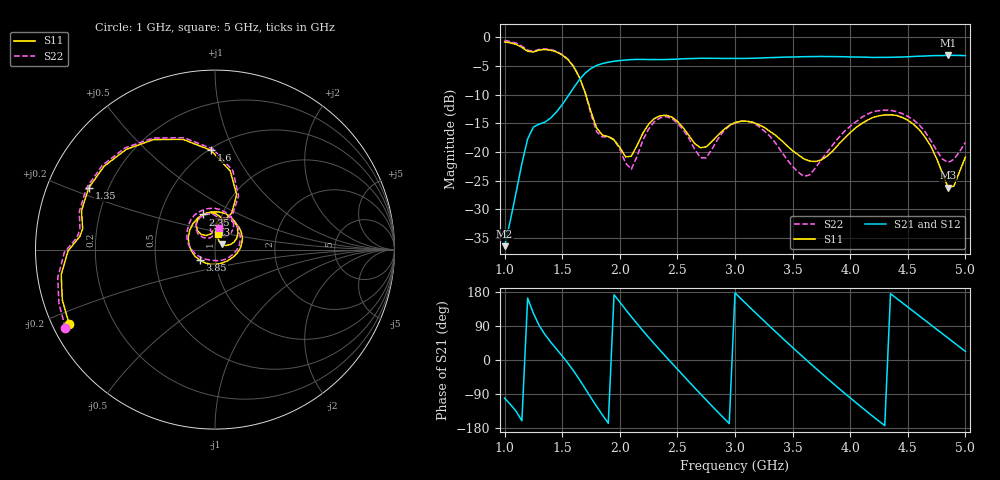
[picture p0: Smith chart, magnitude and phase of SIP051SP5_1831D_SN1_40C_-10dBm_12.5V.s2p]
# GHz  S  dB  R  50
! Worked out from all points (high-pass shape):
!   81 points, 1 GHz to 5 GHz, reference 50 ohm
!   highest |S21| = -3.13 dB at 4.85 GHz (marker M1); lowest = -36.4 dB at 1 GHz (marker M2)
!   |S21| within 3 dB of the highest: 1.706 GHz to end of sweep
!   lowest |S11| = -26.2 dB at 4.85 GHz (marker M3), VSWR 1.10, Z = 54 + j3.19 ohm
!   |S11| at or under -10 dB: 1.705 GHz to end of sweep
!   |S22| runs from -24.3 to -0.5 dB; largest |S21 - S12| = 0.0021
!   S11 on the Smith chart (normalised r, x): 1 GHz: 0.05, -0.24; 1.35 GHz: 0.13, +0.23; 1.6 GHz: 0.51, +0.82; 2.35 GHz: 0.81, +0.33; 3.85 GHz: 0.84, -0.10; 5 GHz: 1.02, +0.18
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1  -0.80 -153.1  -36.42 -100.7  -36.47 -102.9  -0.53 -152.4
1.2  -2.43 174.4  -17.72 163.4  -17.72 163.3  -2.25 175.0
1.35  -2.12 153.9  -14.78 67.2  -14.77 67.1  -2.00 154.2
1.6  -5.14 92.3  -8.76 -29.4  -8.76 -29.4  -5.04 91.1
1.7  -9.67 68.5  -6.22 -75.5  -6.24 -75.5  -9.75 66.2
1.8  -15.85 73.4  -4.88 -123.0  -4.89 -123.1  -16.50 73.3
1.95  -17.89 91.5  -4.16 172.5  -4.18 172.5  -17.82 89.5
2.15  -18.82 132.0  -3.85 95.7  -3.84 95.7  -20.75 133.9
2.35  -13.68 108.9  -3.87 25.5  -3.88 25.5  -14.04 113.9
2.5  -14.62 81.3  -3.80 -24.1  -3.79 -24.3  -14.97 82.8
2.7  -19.25 80.3  -3.64 -89.4  -3.65 -89.5  -20.98 80.8
2.85  -17.07 89.3  -3.66 -137.0  -3.66 -137.0  -17.76 102.4
3  -14.86 69.9  -3.67 177.2  -3.67 177.1  -14.95 79.8
3.3  -16.35 12.5  -3.53 89.3  -3.53 89.3  -17.17 10.9
3.5  -19.77 -28.5  -3.42 33.0  -3.42 32.9  -22.50 -49.5
3.7  -21.65 -88.7  -3.34 -21.7  -3.34 -21.7  -22.71 -131.8
3.85  -19.78 -144.6  -3.33 -61.5  -3.35 -61.5  -18.70 -171.2
4.05  -15.72 155.7  -3.43 -112.5  -3.43 -112.6  -14.71 148.0
4.35  -13.51 84.5  -3.47 174.9  -3.48 174.9  -12.71 92.1
4.6  -16.12 35.2  -3.28 116.3  -3.29 116.3  -15.25 52.8
4.85  -26.22 37.2  -3.13 57.7  -3.15 57.7  -21.83 63.2
5  -20.89 77.9  -3.17 22.9  -3.17 23.0  -18.29 80.5
